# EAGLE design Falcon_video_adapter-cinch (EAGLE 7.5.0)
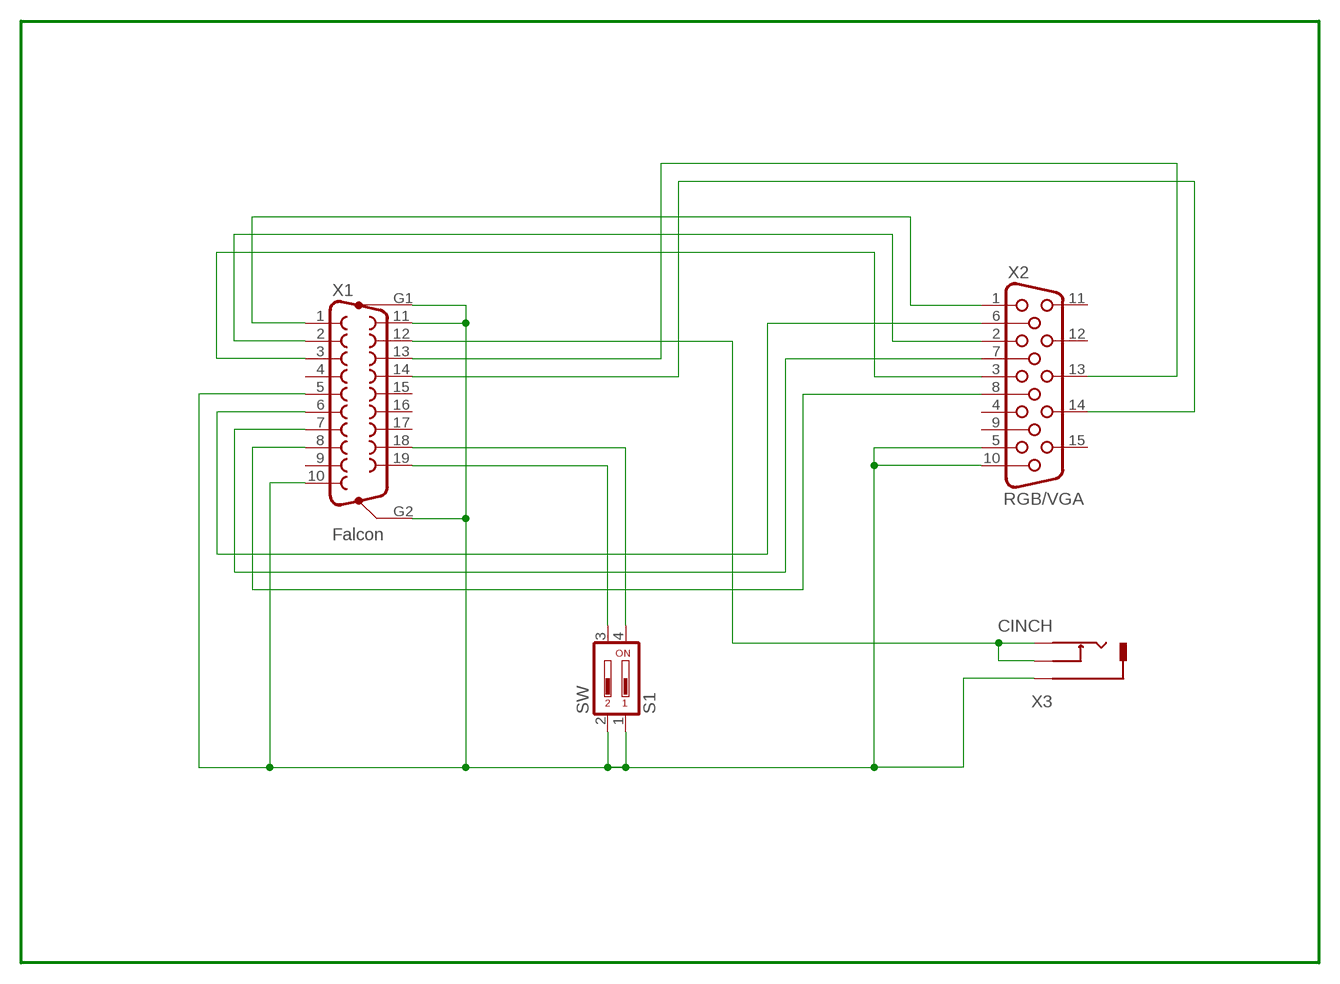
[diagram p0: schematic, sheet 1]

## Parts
S1  SW  DIP02YL  [DIP02YL]
X1  Falcon  F19HP  [F19HP]
X2  RGB/VGA  HF15H  [HDF15H]
X3  CINCH  [SJC-0358]

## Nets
B: X1.3 X2.3
COMPOSITE: X1.12 X3.1 X3.3
G: X1.2 X2.2
GND: S1.1 S1.2 X1.5 X1.10 X1.11 X1.G1 X1.G2 X2.5 X2.10 X3.2
GND_B: X1.8 X2.8
GND_G: X1.7 X2.7
GND_R: X1.6 X2.6
HS: X1.14 X2.14
M0: S1.3 X1.19
M1: S1.4 X1.18
R: X1.1 X2.1
VS: X1.13 X2.13
Unconnected: X1.4 X1.9 X1.15 X1.16 X1.17 X2.4 X2.9 X2.11 X2.12 X2.15

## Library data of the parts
S1 = switch-dil:DIP02YL: DIL/CODE SWITCH; OC_FARNELL: unknown; OC_NEWARK: unknown
X1 = dsub_F19:F19HP: SUB-D; OC_FARNELL: unknown; OC_NEWARK: unknown
X2 = con-subd:HF15: SUB-D; OC_FARNELL: unknown; OC_NEWARK: unknown
X3 = cinch:CINCH: Cinch Connector ( RCA Jack )

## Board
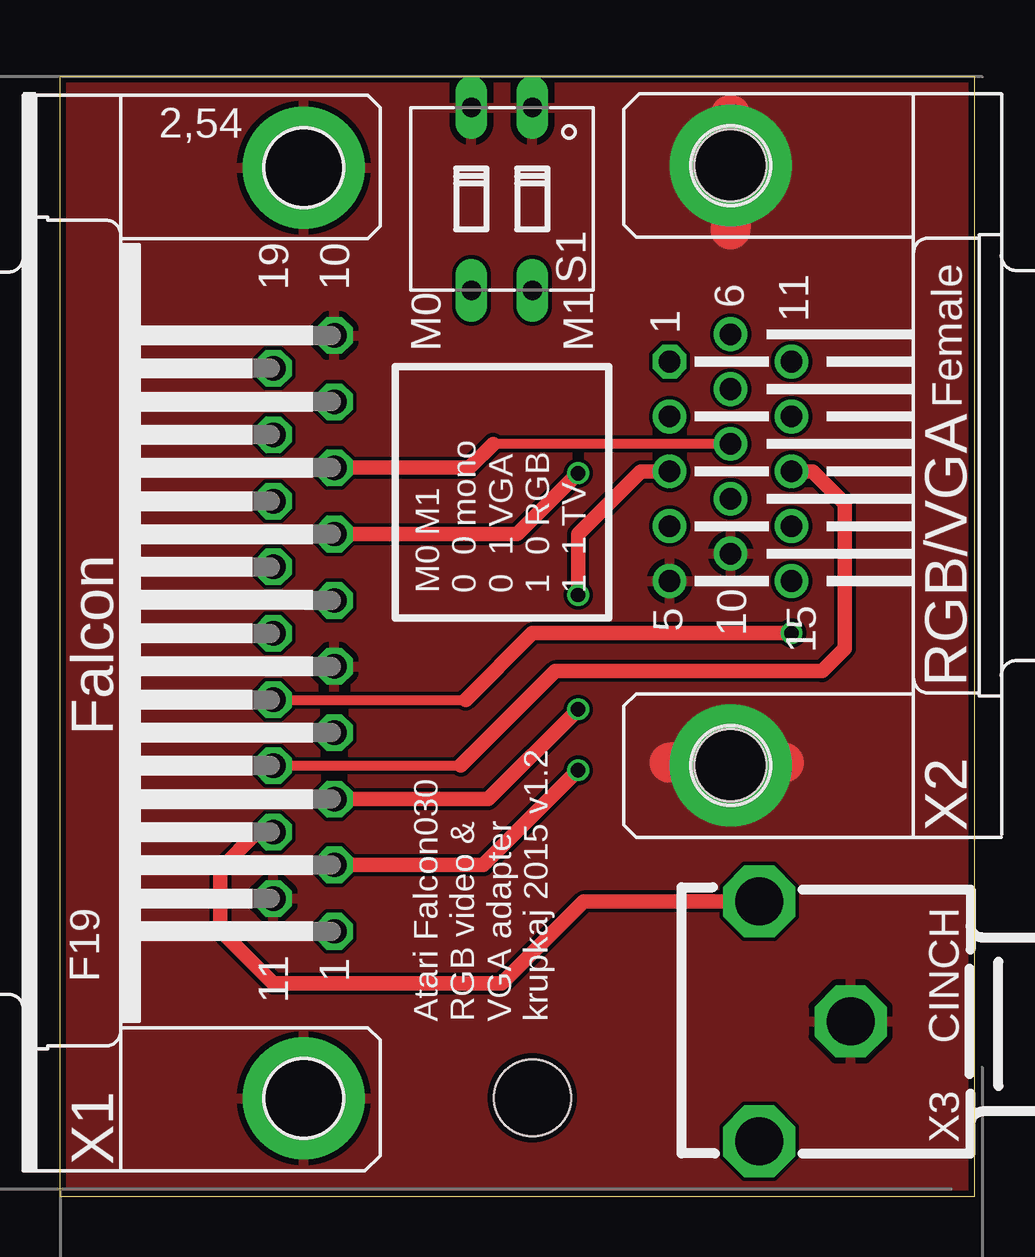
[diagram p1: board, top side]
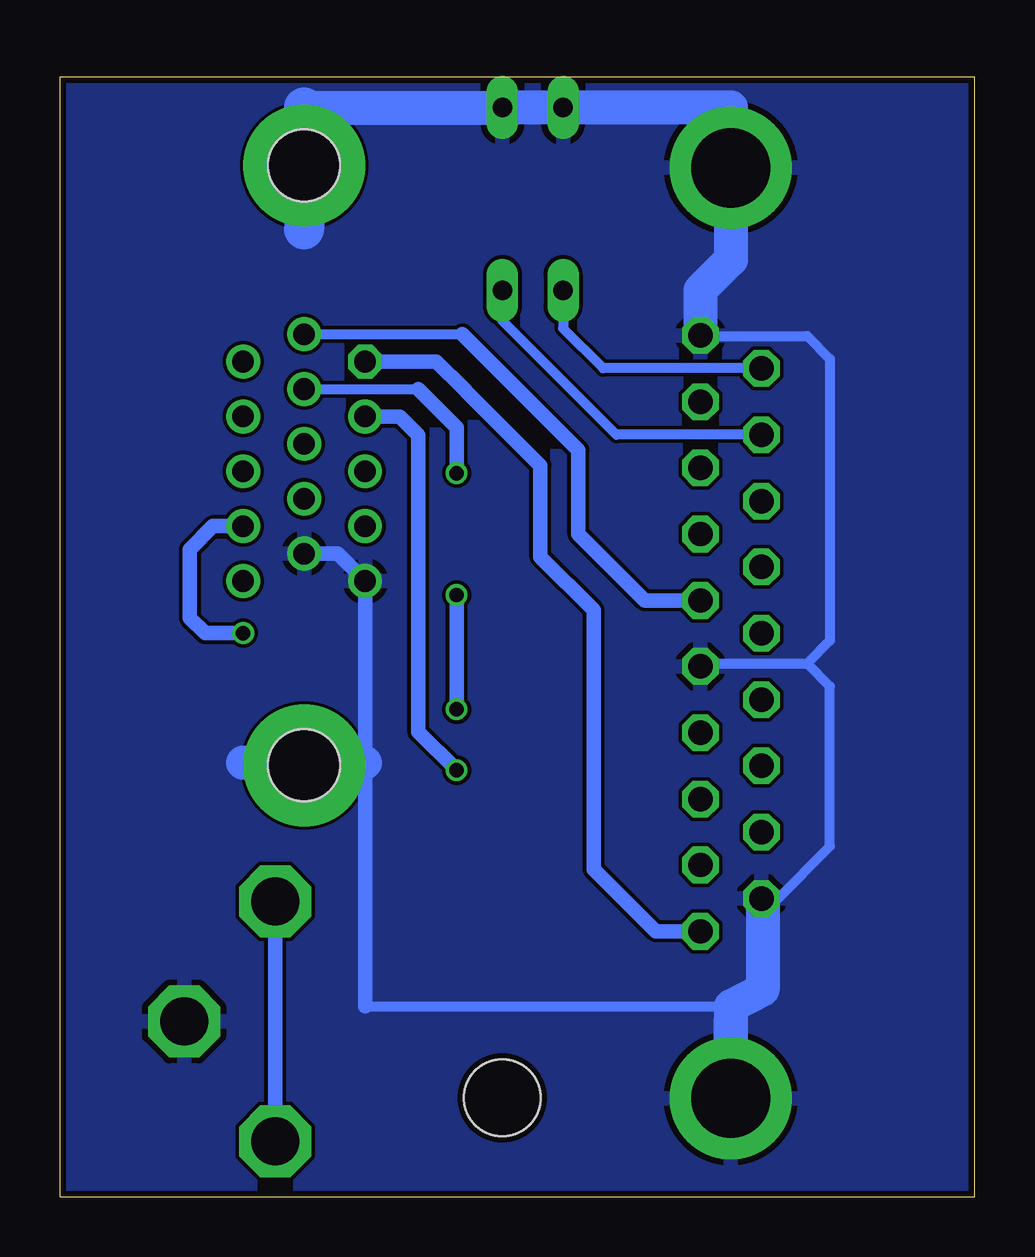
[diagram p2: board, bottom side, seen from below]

Size 38.11 x 46.69 mm. Coordinates in mm from the lower left corner, seen from the top.
Outline: 38.11,0 38.11,46.68 0,46.69 0,0 38.11,0
Copper layers (1*16): Top 0.035mm / dielectric 1.5mm / Bottom 0.035mm
Design rules "SeeedStudio_2layer_DRU_no_angle_20140221": minimum track width 6mil, minimum drill 12mil, track to track 6mil, track to pad 6mil, pad to pad 6mil, via to via 6mil, smd to smd 0mil, copper to edge 10mil, drill to drill 10mil, minimum pad ring 10mil, minimum via ring 6mil, stop-mask expansion 2mil, vias tented up to drill 100mil, thermal gap 10mil
Holes 3.2 mm at 19.69,4.13

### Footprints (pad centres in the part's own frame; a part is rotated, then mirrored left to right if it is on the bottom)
DIP02YL = drill 0.813 long: 1 -1.27,-3.81; 2 1.27,-3.81; 3 1.27,3.81; 4 -1.27,3.81
F19HP = drill 1.016 octagon: 1 -16.561,-1.27; 2 -13.792,-1.27; 3 -11.049,-1.27; 4 -8.28,-1.27; 5 -5.512,-1.27; 6 -2.769,-1.27; 7 0,-1.27; 8 2.769,-1.27; 9 5.512,-1.27; 10 8.28,-1.27; 11 -15.189,1.27; 12 -12.421,1.27; 13 -9.652,1.27; 14 -6.909,1.27; 15 -4.14,1.27; 16 -1.372,1.27; 17 1.372,1.27; 18 4.14,1.27; 19 6.909,1.27 | drill 3.302 pad 5.08: G1 -23.52,0; G2 15.265,0
HDF15H = drill 0.9 octagon: 1 4.329,2.54 | drill 0.9: 2 2.043,2.54; 3 -0.243,2.54; 4 -2.529,2.54; 5 -4.815,2.54; 6 5.472,0; 7 3.186,0; 8 0.9,0; 9 -1.386,0; 10 -3.672,0; 11 4.329,-2.54; 12 2.043,-2.54; 13 -0.243,-2.54; 14 -2.529,-2.54; 15 -4.815,-2.54 | hole 3: -12.5,0; 12.5,0
SJC-0358 = drill 2 octagon: 1 8.96,5; 2 5.16,0; 3 8.96,-5

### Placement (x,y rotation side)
S1  18.41,41.59 180 top
X1  10.16,27.62 90 top
X2  27.94,30.48 90 top
X3  38.1,7.3 180 top

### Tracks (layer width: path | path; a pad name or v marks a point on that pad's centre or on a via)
B  (via drill 0.6)
  Top 0.61: X1.3 17.84,16.57 v21.59,20.32 | v21.59,25.08 21.59,27.62 24.2,30.24 X2.3
  Bottom 0.61: v21.59,20.32 v21.59,25.08
COMPOSITE
  Top 0.61: X1.12 8.22,15.2 6.67,13.65 6.67,11.11 8.89,8.89 18.41,8.89 21.83,12.3 X3.3
  Bottom 0.61: X3.1 X3.3
G  (via drill 0.6)
  Top 0.61: X1.2 17.64,13.83 v21.59,17.78
  Bottom 0.61: v21.59,17.78 23.18,19.37 23.18,31.75 23.95,32.52 X2.2
GND  (via drill 3 pad 5.08)
  Top 1.676: 30.16,18.1 25.4,18.1 | 27.94,45.09 27.94,40.32
  Bottom 0.406: X1.11 8.84,12.38 8.25,12.38 6.03,14.6 6.03,21.27 6.99,22.23 | X1.5 11.32,22.23 6.99,22.23 | X1.10 11.41,35.88 6.99,35.88 6.03,34.92 6.03,23.18 6.99,22.23 | 25.4,7.94 10.16,7.94
  Bottom 0.61: X2.10 26.54,26.81 X2.5 25.4,18.1 25.4,17.97 | 25.4,17.97 v27.94,17.97 | 25.4,17.97 25.4,7.94
  Bottom 1.422: X1.10 11.43,37.78 10.16,39.05 X1.G2 10.16,45.4 S1.2 S1.1 27.94,45.4 v27.94,42.99 | 8.84,12.38 8.84,8.62 10.16,7.94 X1.G1 10.18,7.3 | v27.94,17.97 30.48,18.1 25.4,18.1
  Bottom 1.676: 27.94,45.4 27.94,40.32
  pour Bottom: 38.84,47.97 38.84,-1.26 -0.13,-1.26 -0.13,0.14 -0.41,0.14 -0.41,9.44 0,37.22 -0.23,48.5
  pour Top: -0.2,48.87 38.91,48.87 38.91,-1.26 -0.38,-1.26 -0.38,9.39 -0.18,37.3 -0.18,47.26
GND_B
  Top 0.406: X2.8 18.05,31.38
  Top 0.61: 18.05,31.38 17.06,30.39 X1.8
GND_G  (via drill 0.6)
  Top 0.61: X1.7 19.05,27.62 v21.59,30.16
  Bottom 0.406: X2.7 23.19,33.67
  Bottom 0.61: v21.59,30.16 21.59,32.07 23.19,33.67
GND_R
  Bottom 0.406: X2.6 21.35,35.95
  Bottom 0.61: 21.35,35.95 16.51,31.12 16.51,27.62 13.74,24.85 X1.6
HS  (via drill 0.6)
  Top 0.406: X1.14 16.9,20.71
  Top 0.61: v30.48,23.49 19.69,23.49 16.9,20.71
  Bottom 0.61: X2.14 31.74,27.95 32.7,26.99 32.7,24.13 32.07,23.49 v30.48,23.49
M0
  Bottom 0.406: X1.19 15.48,34.53 17.14,36.2 S1.3
M1
  Bottom 0.406: X1.18 14.94,31.76 19.69,36.51 S1.4
R
  Bottom 0.61: X2.1 22.43,34.81 21.27,33.65 21.11,33.5 18.1,30.48 18.1,26.67 15.88,24.45 15.88,13.65 13.28,11.06 X1.1
VS
  Top 0.406: X1.13 16.7,17.97
  Top 0.61: X2.13 31.36,30.24 32.7,28.89 32.7,22.86 31.75,21.91 20.64,21.91 16.7,17.97

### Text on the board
tNames: M0 | M1 | M0 M1 / 0 0 mono / 0 1 VGA / 1 0 RGB / 1 1 TV | Atari Falcon030 / RGB video & / VGA adapter / krupkaj 2015 v1.2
